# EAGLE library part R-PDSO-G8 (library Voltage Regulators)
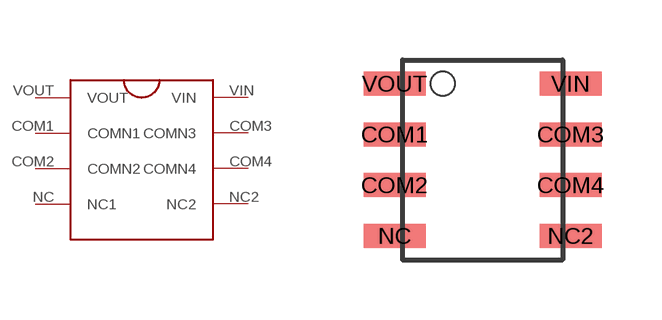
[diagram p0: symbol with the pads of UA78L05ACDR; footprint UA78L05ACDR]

Designator prefix -

## R-PDSO-G8  [UA78L05ACDR]
COM1  COMN1
COM2  COMN2
COM3  COMN3
COM4  COMN4
NC  NC1
NC2  NC2
VIN  VIN
VOUT  VOUT

## Footprint UA78L05ACDR (pad centres in mm)
smd 1.55 x 0.6: COM1 -2.4,0.73; COM2 -2.4,-0.54; COM3 2,0.73; COM4 2,-0.54; NC -2.4,-1.81; NC2 2,-1.81; VIN 2,2; VOUT -2.4,2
